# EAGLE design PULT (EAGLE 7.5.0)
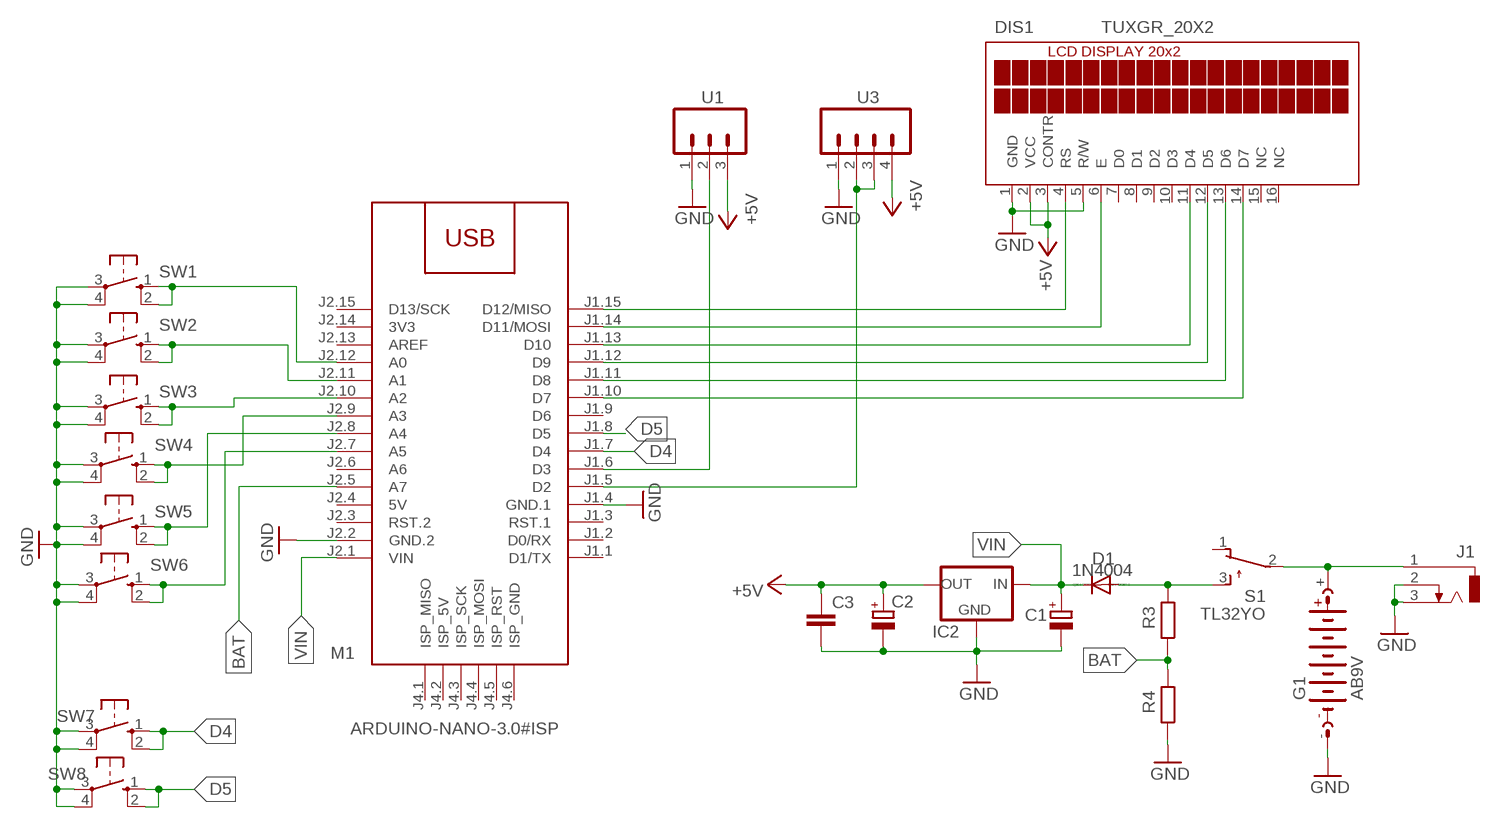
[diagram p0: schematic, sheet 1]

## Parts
C1  CPOL-EUE2.5-6  [E2,5-6]
C2  CPOL-EUE2.5-6  [E2,5-6]
C3  C-EUC1206  [C1206]
D1  1N4004  [DO41-10]
DIS1  TUXGR_20X2  [TUXGR_20X2]
G1  AB9V  [AB9V]
IC2  78XXS  [78XXS]
J1  DCJ0303  [DCJ0303]
M1  ARDUINO-NANO-3.0#ISP  [ARDUINO-NANO-3.0#ISP]
R3  R-EU_0207/10  [0207/10]
R4  R-EU_0207/10  [0207/10]
S1  TL32YO  [TL3XYO]
SW1  40-XX  [B3F-40XX]
SW2  40-XX  [B3F-40XX]
SW3  40-XX  [B3F-40XX]
SW4  40-XX  [B3F-40XX]
SW5  40-XX  [B3F-40XX]
SW6  40-XX  [B3F-40XX]
SW7  40-XX  [B3F-40XX]
SW8  40-XX  [B3F-40XX]
U1  M03  [03P]
U3  M04  [04P]

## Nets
9V: D1.A R3.2 S1.3(S)
+5V: C2.+ C3.1 DIS1.2(VCC) DIS1.3(CONTR) IC2.OUT U1.3 U3.4
BAT: M1.J2.5(A7) R3.1 R4.2
D4: M1.J1.7(D4) SW7.1(S) SW7.2(S1)
D5: M1.J1.8(D5) SW8.1(S) SW8.2(S1)
GND: C1.- C2.- C3.2 DIS1.1(GND) DIS1.5(R/W) G1.- IC2.GND J1.2 J1.3 M1.J1.4(GND.1) M1.J2.2(GND.2) R4.1 SW1.3(P) SW1.4(P1) SW2.3(P) SW2.4(P1) SW3.3(P) SW3.4(P1) SW4.3(P) SW4.4(P1) SW5.3(P) SW5.4(P1) SW6.3(P) SW6.4(P1) SW7.3(P) SW7.4(P1) SW8.3(P) SW8.4(P1) U1.1 U3.1
N$1: M1.J1.6(D3) U1.2
N$2: M1.J1.5(D2) U3.2 U3.3
N$3: M1.J2.12(A0) SW1.1(S) SW1.2(S1)
N$4: M1.J2.8(A4) SW5.1(S) SW5.2(S1)
N$5: DIS1.4(RS) M1.J1.15(D12/MISO)
N$6: DIS1.6(E) M1.J1.14(D11/MOSI)
N$7: DIS1.11(D4) M1.J1.13(D10)
N$8: DIS1.12(D5) M1.J1.12(D9)
N$9: DIS1.13(D6) M1.J1.11(D8)
N$10: DIS1.14(D7) M1.J1.10(D7)
N$11: M1.J2.11(A1) SW2.1(S) SW2.2(S1)
N$12: M1.J2.10(A2) SW3.1(S) SW3.2(S1)
N$13: M1.J2.9(A3) SW4.1(S) SW4.2(S1)
N$14: M1.J2.7(A5) SW6.1(S) SW6.2(S1)
N$34: G1.+ J1.1 S1.2(P)
VIN: C1.+ D1.C IC2.IN M1.J2.1(VIN)
Unconnected: DIS1.7(D0) DIS1.8(D1) DIS1.9(D2) DIS1.10(D3) DIS1.15(NC) DIS1.16(NC) M1.J1.1(D1/TX) M1.J1.2(D0/RX) M1.J1.3(RST.1) M1.J1.9(D6) M1.J2.3(RST.2) M1.J2.6(A6) M1.J2.13(AREF) M1.J2.15(D13/SCK) M1.J4.1(ISP_MISO) M1.J4.2(ISP_5V) M1.J4.3(ISP_SCK) M1.J4.4(ISP_MOSI) M1.J4.5(ISP_RST) M1.J4.6(ISP_GND) S1.1(O)

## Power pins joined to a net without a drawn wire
3V3: M1.J2.14(3V3)
5V: M1.J2.4(5V)

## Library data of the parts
C1 C2 = rcl:CPOL-EU: POLARIZED CAPACITOR, European symbol
C3 = rcl:C-EU: CAPACITOR, European symbol
D1 = diode:1N4004: DIODE
DIS1 = display-lcd:TUXGR_20X2: Tuxgraphics LCD display 20x2 characters reflective, without background light Source: tuxgr_20x2.pdf; OC_FARNELL: unknown; OC_NEWARK: unknown
G1 = battery:AB9V: 9-V BATTERY CLIP
IC2 = v-reg:78XXS: VOLTAGE REGULATOR
J1 = con-jack:DCJ0303: DC POWER JACK Source: DCJ0303.pdf; OC_FARNELL: unknown; OC_NEWARK: unknown
M1 = diy-modules:ARDUINO-NANO-3.0#ISP: Arduino Nano 3.0 (and compatible devices) with ISP pads More details available here: https://www.arduino.cc/en/Main/ArduinoBoardNano Click here to find device on ebay.com
R3 R4 = rcl:R-EU_: RESISTOR, European symbol
S1 = switch:TL32YO: TINY SWITCH ON - MOM Source: http://www2.produktinfo.conrad.com/datenblaetter/700000-724999/705152-da-01-de-Subminiaturschalter_TL_36YO.pdf
SW1-SW8 = switch-omron:40-XX: OMRON SWITCH; MF: OMRON COMPONENTS USA; MPN: B3F-4000; OC_FARNELL: 176434; OC_NEWARK: 36K3105
U1 = con-amp-quick:M03: AMP QUICK CONNECTOR; OC_FARNELL: unknown; OC_NEWARK: unknown
U3 = con-amp-quick:M04: AMP QUICK CONNECTOR; OC_FARNELL: unknown; OC_NEWARK: unknown

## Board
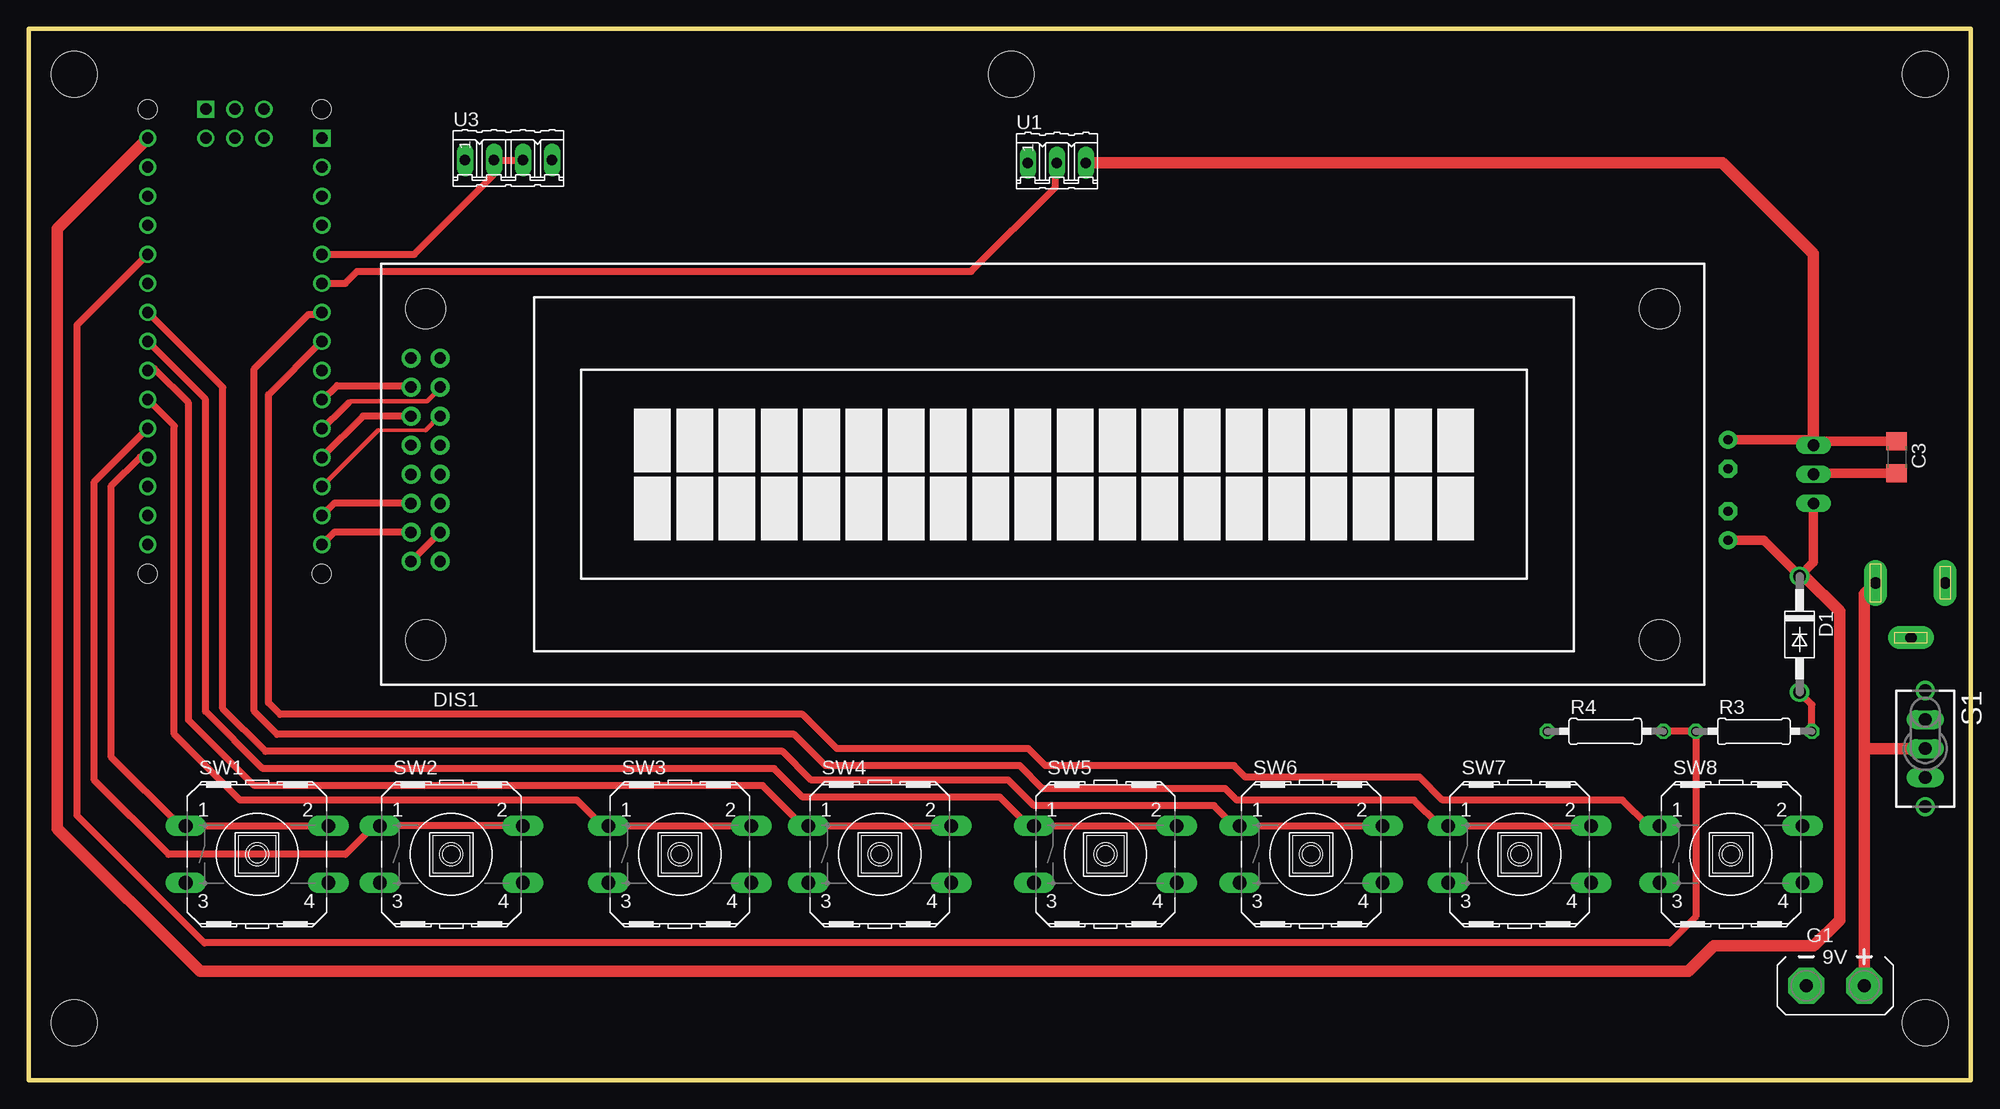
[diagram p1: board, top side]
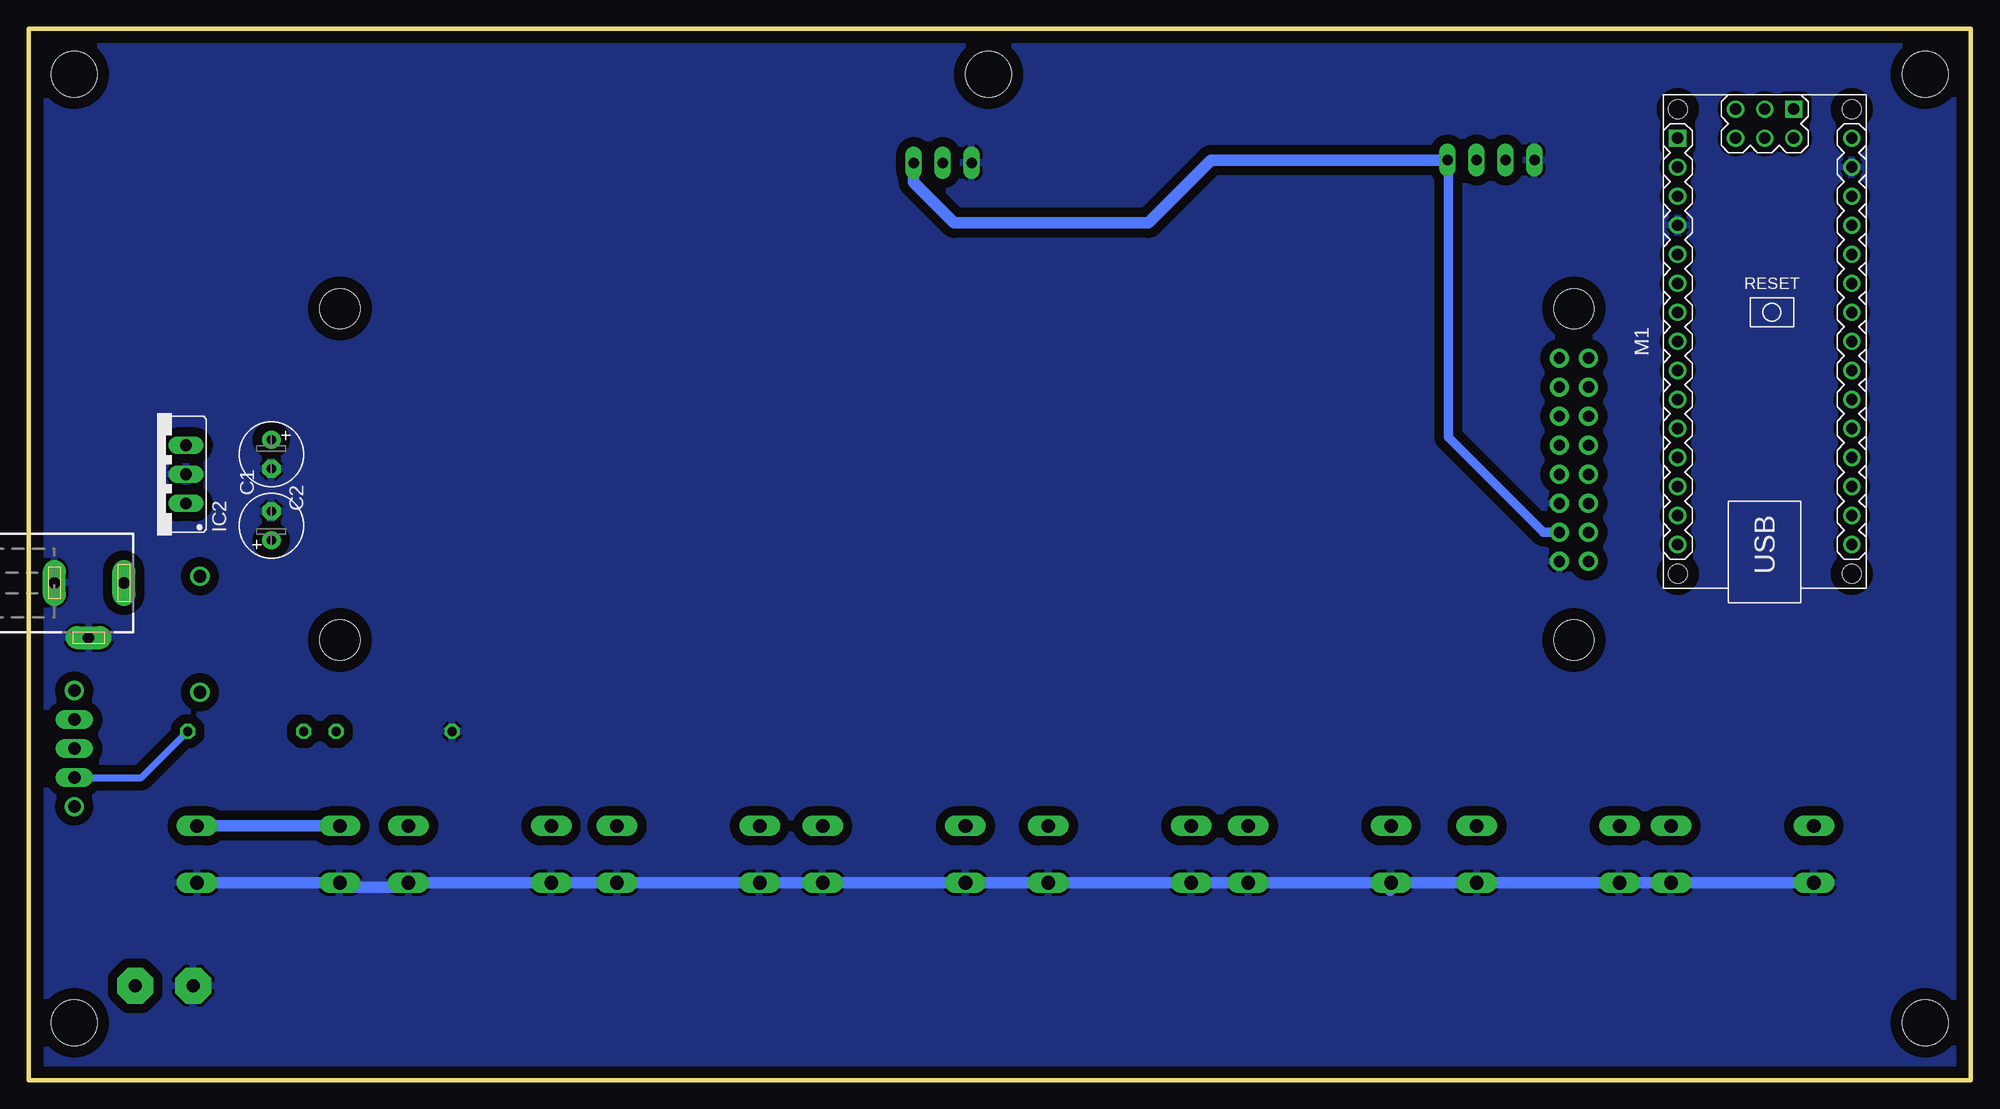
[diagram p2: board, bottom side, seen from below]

Size 170 x 92 mm. Coordinates in mm from the lower left corner, seen from the top.
Outline: 0,0 0,92 170,92 170,0 0,0
Copper layers (1*16): Top 0.035mm / dielectric 1.5mm / Bottom 0.035mm
Design rules "default": minimum track width 10mil, minimum drill 24mil, track to track 8mil, track to pad 8mil, pad to pad 8mil, via to via 8mil, smd to smd 8mil, copper to edge 40mil, drill to drill 8mil, minimum pad ring 10mil, minimum via ring 8mil, stop-mask expansion 4mil, vias tented up to drill 0mil, thermal gap 10mil
Holes 4 mm at 4,5 166,5 4,88 166,88 86,88

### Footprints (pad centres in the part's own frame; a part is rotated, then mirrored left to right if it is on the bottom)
E2,5-6 = drill 0.813 pad 1.6: + -1.27,0 | drill 0.813 pad 1.6 octagon: - 1.27,0
C1206 = smd 1.6 x 1.8: 1 -1.4,0; 2 1.4,0
DO41-10 = drill 1.118: A 5.08,0; C -5.08,0
TUXGR_20X2 = drill 1 pad 1.676: 1 -52.73,-7.62; 2 -55.27,-7.62; 3 -52.73,-5.08; 4 -55.27,-5.08; 5 -52.73,-2.54; 6 -55.27,-2.54; 7 -52.73,0; 8 -55.27,0; 9 -52.73,2.54; 10 -55.27,2.54; 11 -52.73,5.08; 12 -55.27,5.08; 13 -52.73,7.62; 14 -55.27,7.62; 15 -52.73,10.16; 16 -55.27,10.16 | hole 3.5: -54,-14.5; 54,-14.5; -54,14.5; 54,14.5
AB9V = drill 1.118 pad 3.15 octagon: + 0,2.54; - 0,-2.54
78XXS = drill 1.016 long: GND 0,-2.54; IN -2.54,-2.54; OUT 2.54,-2.54
DCJ0303 = drill 1 pad 2 long: 1 0,3.1; 2 4.8,0; 3 0,-3
ARDUINO-NANO-3.0#ISP = drill 1 square: J1.1 17.78,7.62; J4.1 20.32,-2.54 | drill 1: J1.2 15.24,7.62; J1.3 12.7,7.62; J1.4 10.16,7.62; J1.5 7.62,7.62; J1.6 5.08,7.62; J1.7 2.54,7.62; J1.8 0,7.62; J1.9 -2.54,7.62; J1.10 -5.08,7.62; J1.11 -7.62,7.62; J1.12 -10.16,7.62; J1.13 -12.7,7.62; J1.14 -15.24,7.62; J1.15 -17.78,7.62; J2.1 17.78,-7.62; J2.2 15.24,-7.62; J2.3 12.7,-7.62; J2.4 10.16,-7.62; J2.5 7.62,-7.62; J2.6 5.08,-7.62; J2.7 2.54,-7.62; J2.8 0,-7.62; J2.9 -2.54,-7.62; J2.10 -5.08,-7.62; J2.11 -7.62,-7.62; J2.12 -10.16,-7.62; J2.13 -12.7,-7.62; J2.14 -15.24,-7.62; J2.15 -17.78,-7.62; J4.2 17.78,-2.54; J4.3 20.32,0; J4.4 17.78,0; J4.5 20.32,2.54; J4.6 17.78,2.54 | hole 1.651: -20.32,7.62; -20.32,-7.62; 20.32,-7.62; 20.32,7.62
0207/10 = drill 0.813 octagon: 1 -5.08,0; 2 5.08,0
TL3XYO = drill 1.1 pad 1.422 long: 1 -2.54,0; 2 0,0; 3 2.54,0 | drill 1.1 pad 1.676: M1 -5.08,0; M2 5.08,0
B3F-40XX = drill 1.194 long: 1 -6.248,2.489; 2 6.248,2.489; 3 -6.248,-2.489; 4 6.248,-2.489
03P = drill 0.914 long: 1 -2.54,0; 2 0,0; 3 2.54,0
04P = drill 0.914 long: 1 -3.81,0; 2 -1.27,0; 3 1.27,0; 4 3.81,0

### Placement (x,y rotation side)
C1  148.75,48.5 90 bottom
C2  148.75,54.75 270 bottom
C3  163.5,54.5 270 top
D1  155,39 270 top
DIS1  88.75,53 0 top
G1  158.12,8.25 270 top
IC2  158.75,53 90 bottom
J1  164.75,43.5 270 bottom
M1  18.05,64.63 90 bottom
R3  151,30.5 0 top
R4  138,30.5 0 top
S1  166,29 270 top
SW1  20,19.75 0 top
SW2  37,19.75 0 top
SW3  57,19.75 0 top
SW4  74.5,19.75 0 top
SW5  94.25,19.75 0 top
SW6  112.25,19.75 0 top
SW7  130.5,19.75 0 top
SW8  149,19.75 0 top
U1  90,80.25 0 top
U3  42,80.5 0 top

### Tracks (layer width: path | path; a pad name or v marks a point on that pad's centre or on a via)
9V
  Top 0.61: R3.2 156.08,32.84 D1.A
  Bottom 0.61: S1.3 160.12,26.46 R3.2
+5V
  Top 0.61: DIS1.3 DIS1.2
  Top 0.813: C2.+ 155.73,56.02 IC2.OUT 156.57,55.9 C3.1
  Top 1.016: IC2.OUT 156.21,72.29 148.25,80.25 U1.3
  Bottom 0.813: DIS1.3 37.42,47.92 45.75,56.25 45.75,80.44 U3.4
  Bottom 1.016: U3.4 66.5,80.5 72,75 89,75 92.54,78.54 U1.3
BAT
  Top 0.61: M1.J2.5 4.25,66.07 4.25,23.12 15.38,12 143.62,12 145.92,14.29 R3.1 R4.2
D4
  Top 0.61: SW7.2 SW7.1 123.51,22.24 121.25,24.5 105.75,24.5 104.75,25.5 88.75,25.5 86.75,27.5 69.75,27.5 67,30.25 21.75,30.25 19.75,32.25 19.75,62.25 24.5,67 25.5,67 M1.J1.7
D5
  Top 0.61: SW8.1 141.76,22.24 139.5,24.5 123.75,24.5 121.75,26.5 106.5,26.5 105.5,27.5 89,27.5 87.5,29 70.75,29 67.75,32 22,32 21,33 21,59.96 M1.J1.8
  Bottom 1.016: SW8.1 SW8.2
GND
  Top 0.813: C3.2 156.31,53.1 IC2.GND
  Bottom 1.016: SW1.3 SW1.4 SW2.3 SW2.4 50.24,17.26 50.88,16.62 50.88,17.14 SW3.3 SW3.4 SW4.3 SW4.4 SW5.3 SW5.4 SW6.3 SW6.4 SW7.3 SW7.4 137.61,17.26 138,16.88 142.37,16.88 SW8.3 154.49,17.26 154.62,17.12 155.11,17.12 SW8.4
  pour Bottom (isolate 0.813): 1,91 169,91 169,1 1,1
N$1
  Top 0.61: M1.J1.6 27.71,69.71 28.75,70.75 82.5,70.75 89.88,78.12 89.88,80.12 U1.2
N$2
  Top 0.61: M1.J1.5 33.75,72.25 40.62,79.12 40.62,80.39 U3.2 U3.3
N$3
  Top 0.61: M1.J2.12 10.4,54.5 9.75,54.5 7.25,52 7.25,28.25 13.26,22.24 SW1.1 SW1.2
N$4
  Top 0.61: M1.J2.8 15.5,59.56 15.5,32.25 20.5,27.25 65.25,27.25 67.75,24.75 85,24.75 87.51,22.24 SW5.1 SW5.2
N$5
  Top 0.61: DIS1.4 26.74,47.92 M1.J1.15
N$6
  Top 0.61: DIS1.6 26.74,50.46 M1.J1.14
N$7
  Top 0.305: 34.75,56.88 30.61,56.88
  Top 0.406: DIS1.11 35.95,58.08 34.75,56.88 | 30.61,56.88 M1.J1.13
N$8
  Top 0.61: DIS1.12 29.28,58.08 M1.J1.12
N$9
  Top 0.406: DIS1.13 36.02,60.52 34.88,59.38 28.12,59.38 27.56,58.81
  Top 0.61: M1.J1.11 25.76,57.01 27.56,58.81 28,59.25
N$10
  Top 0.61: M1.J1.10 25.8,59.55 27,60.75 33.35,60.75 DIS1.14
N$11
  Top 0.61: M1.J2.11 5.75,52.33 5.75,26.25 12.25,19.75 27.75,19.75 30.24,22.24 SW2.1 SW2.2
N$12
  Top 0.61: M1.J2.10 12.75,57.23 12.75,30.25 18.5,24.5 48,24.5 50.26,22.24 SW3.1 SW3.2
N$13
  Top 0.61: M1.J2.9 10.59,62.25 11,62.25 14,59.25 14,31.5 19.75,25.75 64.25,25.75 67.76,22.24 SW4.1 SW4.2
N$14
  Top 0.61: M1.J2.7 17,60.6 17,32.5 20.75,28.75 66,28.75 68.5,26.25 85.75,26.25 88,24 103.75,24 105.51,22.24 SW6.1 SW6.2
N$34
  Top 1.016: G1.+ 160.66,29.25 | 160.66,29.25 160.66,42.52 J1.1 | S1.2 160.91,29 160.66,29.25
VIN
  Top 0.813: IC2.IN 156.21,45.29 D1.C 151.85,47.23 C1.+
  Top 1.016: D1.C 155.42,44.08 158.5,41 158.5,14 156.25,11.75 147.5,11.75 145.25,9.5 15,9.5 2.5,22 2.5,74.48 M1.J2.1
